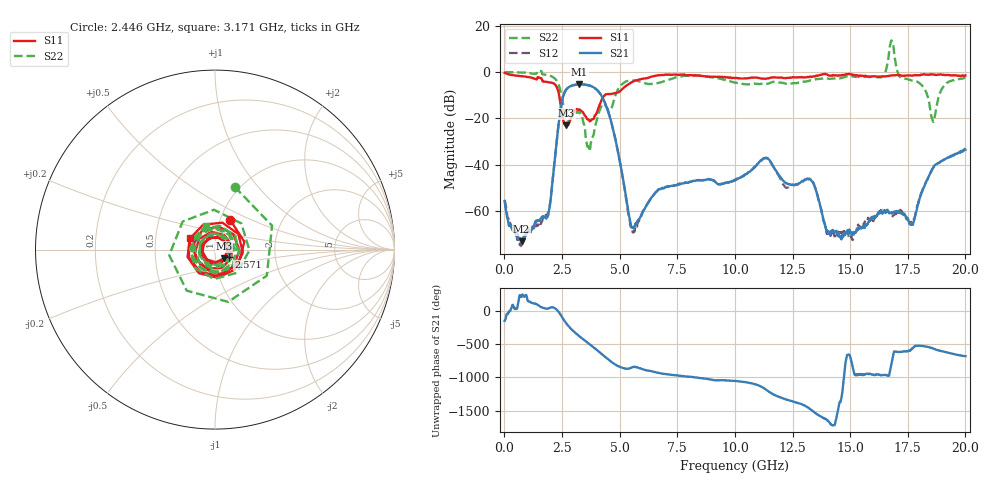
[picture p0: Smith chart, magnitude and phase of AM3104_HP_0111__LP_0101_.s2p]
!Created with skrf (http://scikit-rf.org).
# Hz S RI R 50.0
!freq ReS11 ImS11 ReS21 ImS21 ReS12 ImS12 ReS22 ImS22
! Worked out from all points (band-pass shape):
!   1601 points, 10 MHz to 20 GHz, reference 50 ohm
!   highest |S21| = -5.30 dB at 3.246 GHz (marker M1); lowest = -73.1 dB at 747.1 MHz (marker M2)
!   |S21| within 3 dB of the highest: 2.637 GHz to 4.079 GHz (1.442 GHz wide, 42.9 % of centre)
!   lowest |S11| = -23.1 dB at 2.684 GHz (marker M3), VSWR 1.15, Z = 55 - j5.45 ohm
!   |S11| at or under -10 dB: 2.375 GHz to 4.353 GHz (1.978 GHz wide, 58.8 % of centre)
!   |S22| runs from -34.2 to 13.6 dB; largest |S21 - S12| = 0.029
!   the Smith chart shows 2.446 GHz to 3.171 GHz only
!   S11 on the Smith chart (normalised r, x): 2.446 GHz: 1.12, +0.38; 2.571 GHz: 1.16, -0.10; 3.171 GHz: 0.75, +0.10
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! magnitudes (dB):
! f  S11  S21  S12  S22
! 10 MHz  -0.4  -55.6  -55.2  0.0
! 747.1 MHz  -1.8  -73.1  -74.7  -0.3
! 1.897 GHz  -4.3  -61.9  -60.9  -1.4
! 2.446 GHz  -14.6  -15.5  -15.6  -8.7
! 2.571 GHz  -21.3  -9.9  -9.9  -15.0
! 2.684 GHz  -23.1  -7.6  -7.5  -20.1
! 3.171 GHz  -16.2  -5.4  -5.5  -17.2
! 3.246 GHz  -16.4  -5.3  -5.4  -17.6
! 3.346 GHz  -16.8  -5.3  -5.4  -18.4
! 3.671 GHz  -20.7  -5.8  -5.9  -32.9
! 4.445 GHz  -9.5  -15.3  -15.3  -15.3
! 5.557 GHz  -4.2  -67.2  -68.9  -3.7
! 6.682 GHz  -1.4  -50.8  -50.5  -4.8
! 10.01 GHz  -2.7  -46.7  -46.9  -4.6
! 11.33 GHz  -2.9  -37.1  -37.3  -5.1
! 13.34 GHz  -2.1  -47.1  -47.1  -3.6
! 14.07 GHz  -1.4  -68.9  -70.5  -2.9
! 16.35 GHz  -1.9  -60.6  -59.5  -2.3
! 16.68 GHz  -1.6  -60.6  -60.5  7.2
! 17.69 GHz  -1.6  -65.7  -65.6  -3.7
! 18.59 GHz  -1.0  -41.5  -41.5  -21.1
! 20 GHz  -1.5  -33.5  -33.2  -2.5
